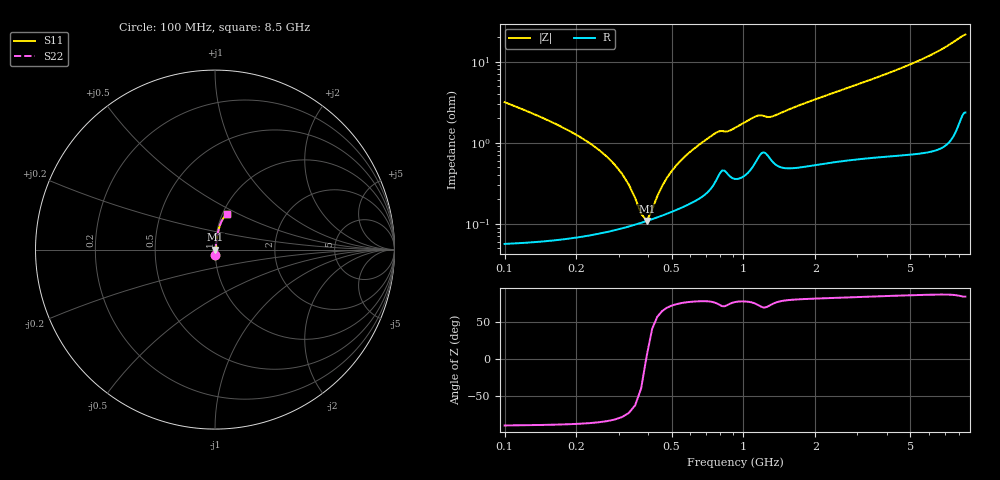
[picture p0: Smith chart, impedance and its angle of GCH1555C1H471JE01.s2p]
!Murata Part Number: GCH1555C1H471JE01
!These Parameters are Measured in Series Mode Connection
!Data Generated on Mar 13, 2026
!  o--ll--o
!Port1  Port2
!  o------o
!Operation Temp=25[degC], DC Bias Voltage=0[V]
!Freq. Start=100[MHz] Stop=9[GHz] 401[Steps]
# Hz S RI R 50
!Freq.(Hz) S11(Real) S11(Imag) S21(Real) S21(Imag) S12(Real) S12(Imag) S22(Real) S22(Imag)
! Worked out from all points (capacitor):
!   401 points, 100 MHz to 8.5 GHz, reference 50 ohm
!   read as one part in series: C = 471 pF near 142 MHz
!   lowest |Z| = 109 mohm at 394 MHz (marker M1)
!   series resonance near 391.8 MHz, so ESL is about 350 pH
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1e8  0.00156 -0.0316  0.9984 0.0316  0.9984 0.0316  0.00156 -0.0316
1.42e8  0.00103 -0.0207  0.999 0.0207  0.999 0.0207  0.00103 -0.0207
2.47e8  0.000823 -0.00822  0.9992 0.00822  0.9992 0.00822  0.000823 -0.00822
2.89e8  0.000864 -0.00531  0.9991 0.00531  0.9991 0.00531  0.000864 -0.00531
3.52e8  0.000981 -0.00184  0.999 0.00184  0.999 0.00184  0.000981 -0.00184
3.73e8  0.00103 -0.000841  0.999 0.000841  0.999 0.000841  0.00103 -0.000841
3.94e8  0.00109 9.84e-05  0.9989 -9.84e-05  0.9989 -9.84e-05  0.00109 9.84e-05
4.15e8  0.00114 0.000989  0.9989 -0.000989  0.9989 -0.000989  0.00114 0.000989
4.78e8  0.00134 0.00343  0.9987 -0.00343  0.9987 -0.00343  0.00134 0.00343
5.41e8  0.00158 0.00563  0.9984 -0.00563  0.9984 -0.00563  0.00158 0.00563
6.25e8  0.00197 0.00834  0.998 -0.00834  0.998 -0.00834  0.00197 0.00834
7.51e8  0.00319 0.0123  0.9968 -0.0123  0.9968 -0.0123  0.00319 0.0123
8.98e8  0.00385 0.014  0.9961 -0.014  0.9961 -0.014  0.00385 0.014
1.129e9  0.00625 0.0202  0.9937 -0.0202  0.9937 -0.0202  0.00625 0.0202
1.318e9  0.0063 0.02  0.9937 -0.02  0.9937 -0.02  0.0063 0.02
1.507e9  0.00541 0.0241  0.9946 -0.0241  0.9946 -0.0241  0.00541 0.0241
2.074e9  0.00658 0.0348  0.9934 -0.0348  0.9934 -0.0348  0.00658 0.0348
2.914e9  0.00862 0.0496  0.9914 -0.0496  0.9914 -0.0496  0.00862 0.0496
4.3e9  0.0126 0.0755  0.9874 -0.0755  0.9874 -0.0755  0.0126 0.0755
5.707e9  0.0191 0.1068  0.9809 -0.1068  0.9809 -0.1068  0.0191 0.1068
7.114e9  0.0321 0.1483  0.9679 -0.1483  0.9679 -0.1483  0.0321 0.1483
8.5e9  0.0642 0.1962  0.9358 -0.1962  0.9358 -0.1962  0.0642 0.1962
